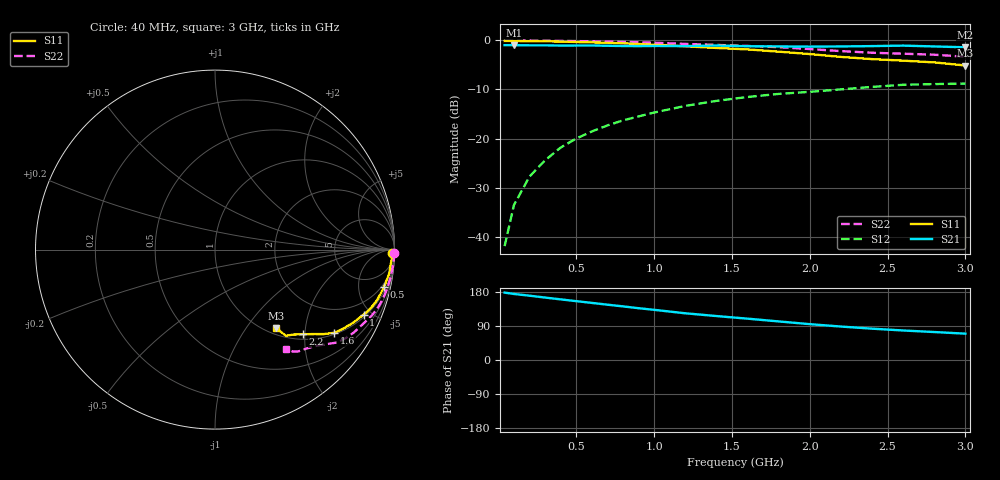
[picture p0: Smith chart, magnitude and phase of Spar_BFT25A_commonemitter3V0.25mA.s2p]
! Filename:  BFT25AG.S2P  Version:  2.0
! NXP part #: BFT25A  Date: Aug 1990
! Bias condition: Vce=3V, Ic=0.25mA
#  MHz  S  MA  R  50
! Freq  S11  S21  S12  S22  !GUM [dB]
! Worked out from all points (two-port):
!   21 points, 40 MHz to 3 GHz, reference 50 ohm
!   highest |S21| = -0.96 dB at 100 MHz (marker M1); lowest = -1.4 dB at 3 GHz (marker M2)
!   |S21| within 3 dB of the highest: start of sweep to end of sweep
!   lowest |S11| = -5.1 dB at 3 GHz (marker M3), VSWR 3.49, Z = 55.3 - j69.9 ohm
!   |S11| at or under -10 dB: nowhere
!   |S22| runs from -3.3 to 0.0 dB; largest |S21 - S12| = 0.9
!   S11 on the Smith chart (normalised r, x): 40 MHz: 48, -71; 500 MHz: 1.50, -8.88; 1 GHz: 1.14, -4.51; 1.6 GHz: 1.05, -2.83; 2.2 GHz: 1.11, -1.95; 3 GHz: 1.11, -1.40
40  0.987 -1.1  0.895 177.8  0.008 86.0  0.999 -1.0
100  0.987 -2.6  0.895 174.3  0.021 86.6  0.998 -2.5
200  0.982 -5.1  0.891 169.7  0.041 85.2  0.996 -5.0
300  0.98 -7.7  0.891 164.8  0.06 83.4  0.992 -7.4
400  0.972 -10.1  0.886 160.0  0.081 81.5  0.989 -9.9
500  0.964 -12.5  0.887 155.3  0.1 79.7  0.984 -12.3
600  0.955 -14.9  0.888 150.7  0.118 77.7  0.979 -14.6
700  0.946 -17.3  0.882 146.0  0.136 75.9  0.973 -16.8
800  0.934 -19.4  0.877 141.5  0.153 74.1  0.966 -18.9
900  0.92 -21.6  0.875 136.7  0.168 72.2  0.957 -20.9
1000  0.904 -23.6  0.878 132.4  0.184 70.2  0.947 -22.9
1200  0.871 -27.9  0.876 123.3  0.215 66.3  0.921 -27.0
1400  0.838 -31.8  0.887 116.0  0.242 63.0  0.9 -31.0
1600  0.81 -34.9  0.872 109.1  0.265 60.1  0.878 -34.3
1800  0.768 -37.8  0.869 101.8  0.285 57.5  0.854 -37.3
2000  0.726 -40.4  0.864 94.6  0.299 53.9  0.817 -40.1
2200  0.679 -44.0  0.868 88.3  0.317 50.8  0.778 -43.6
2400  0.645 -47.2  0.875 82.7  0.336 48.1  0.749 -47.5
2600  0.622 -50.5  0.885 77.9  0.353 46.2  0.732 -50.9
2800  0.597 -51.1  0.868 73.8  0.359 44.8  0.715 -52.6
3000  0.555 -52.1  0.851 69.5  0.363 43.4  0.682 -54.3
